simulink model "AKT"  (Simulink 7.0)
settings: Solver=ode45  StartTime=0.0  StopTime=100  RelTol=1e-3

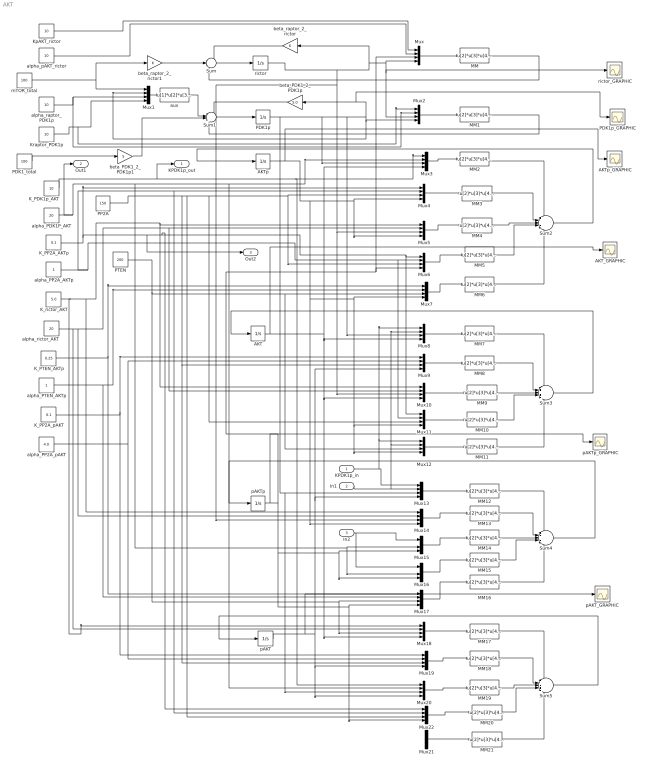
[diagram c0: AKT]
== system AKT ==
  KPDK1p_in : Inport  OutDataType=sfix(16)  OutScaling=2^0
  In1 : Inport  Port=2  OutDataType=sfix(16)  OutScaling=2^0
  In2 : Inport  Port=3  OutDataType=sfix(16)  OutScaling=2^0
  AKT : Integrator  InitialCondition=100.0
  AKT_GRAPHIC : Scope
  AKTp : Integrator  InitialCondition=0.0
  AKTp_GRAPHIC : Scope
  K_PDK1p_AKT : Constant  Value=10  OutDataType=sfix(16)  OutScaling=2^0
  K_PP2A_AKTp : Constant  Value=0.1  OutDataType=sfix(16)  OutScaling=2^0
  K_PP2A_pAKT : Constant  Value=0.1  OutDataType=sfix(16)  OutScaling=2^0
  K_PTEN_AKTp : Constant  Value=0.25  OutDataType=sfix(16)  OutScaling=2^0
  K_rictor_AKT : Constant  Value=5.0  OutDataType=sfix(16)  OutScaling=2^0
  KpAKT_rictor : Constant  Value=10  OutDataType=sfix(16)  OutScaling=2^0
  Kraptor_PDK1p : Constant  Value=10  OutDataType=sfix(16)  OutScaling=2^0
  MM{,1..21} (22 alike) : Fcn  Expr=u[2]*u[3]*u[4]/(u[1]+u[4])
  Mux{,1..22} (23 alike) : Mux
  PDK1_total : Constant  Value=100  OutDataType=sfix(16)  OutScaling=2^0
  PDK1p : Integrator  InitialCondition=50.0
  PDK1p_GRAPHIC : Scope
  PP2A : Constant  Value=150  OutDataType=sfix(16)  OutScaling=2^0
  PTEN : Constant  Value=200  OutDataType=sfix(16)  OutScaling=2^0
  Sum : Sum  Inputs=-+-  OutDataType=sfix(16)  OutScaling=2^0
  Sum1 : Sum  Inputs=--++  OutDataType=sfix(16)  OutScaling=2^0
  Sum2 : Sum  Inputs=+--+-  OutDataType=sfix(16)  OutScaling=2^0
  Sum3 : Sum  Inputs=-+-++  OutDataType=sfix(16)  OutScaling=2^0
  Sum4 : Sum  Inputs=++---  OutDataType=sfix(16)  OutScaling=2^0
  Sum5 : Sum  Inputs=+--++  OutDataType=sfix(16)  OutScaling=2^0
  alpha_PDK1P_AKT : Constant  Value=20  OutDataType=sfix(16)  OutScaling=2^0
  alpha_PP2A_AKTp : Constant  OutDataType=sfix(16)  OutScaling=2^0
  alpha_PP2A_pAKT : Constant  Value=4.0  OutDataType=sfix(16)  OutScaling=2^0
  alpha_PTEN_AKTp : Constant  OutDataType=sfix(16)  OutScaling=2^0
  alpha_pAKT_rictor : Constant  Value=10  OutDataType=sfix(16)  OutScaling=2^0
  alpha_raptor_PDK1p : Constant  Value=10  OutDataType=sfix(16)  OutScaling=2^0
  alpha_rictor_AKT : Constant  Value=20  OutDataType=sfix(16)  OutScaling=2^0
  aux : Fcn  Expr=u[1]*u[2]*u[3]/(u[4]+u[2])
  beta_PDK1_2_PDK1p : Gain  Orientation=left  Gain=5.0  ParameterDataType=sfix(16)  ParameterScaling=2^0  OutDataType=sfix(16)  OutScaling=2^0
  beta_PDK1_2_PDK1p1 : Gain  Gain=5  ParameterDataType=sfix(16)  ParameterScaling=2^0  OutDataType=sfix(16)  OutScaling=2^0
  beta_raptor_2_rictor : Gain  Orientation=left  ParameterDataType=sfix(16)  ParameterScaling=2^0  OutDataType=sfix(16)  OutScaling=2^0
  beta_raptor_2_rictor1 : Gain  ParameterDataType=sfix(16)  ParameterScaling=2^0  OutDataType=sfix(16)  OutScaling=2^0
  mTOR_total : Constant  Value=100  OutDataType=sfix(16)  OutScaling=2^0
  pAKT : Integrator  InitialCondition=.0
  "pAKT_GRAPHIC " : Scope
  pAKTp : Integrator  InitialCondition=0.0
  pAKTp_GRAPHIC : Scope
  rictor : Integrator  InitialCondition=0.0
  rictor_GRAPHIC : Scope
  KPDK1p_out : Outport  OutDataType=sfix(16)  OutScaling=2^0
  Out1 : Outport  Port=2  OutDataType=sfix(16)  OutScaling=2^0
  Out2 : Outport  Port=3  OutDataType=sfix(16)  OutScaling=2^0
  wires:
  Sum/1 -> rictor/1
  rictor/1 -> beta_raptor_2_rictor/1, Mux/4, Mux2/3, rictor_GRAPHIC/1, Mux5/3, Mux10/3, Mux14/3
  beta_raptor_2_rictor/1 -> Sum/1
  beta_raptor_2_rictor1/1 -> Sum/2
  mTOR_total/1 -> beta_raptor_2_rictor1/1, Mux1/1
  Mux/1 -> MM/1
  pAKTp/1 -> Mux/3, Mux6/4, Mux15/4, Mux16/4, Mux17/4, Mux22/4, pAKTp_GRAPHIC/1
  KpAKT_rictor/1 -> Mux/1
  alpha_pAKT_rictor/1 -> Mux/2
  MM/1 -> Sum/3
  Sum1/1 -> PDK1p/1
  PDK1p/1 -> Mux3/3, Mux1/2, Mux2/4, beta_PDK1_2_PDK1p/1, PDK1p_GRAPHIC/1, Mux8/3, Mux13/3, Mux20/3
  beta_PDK1_2_PDK1p/1 -> Sum1/1
  Mux1/1 -> aux/1
  aux/1 -> Sum1/2
  alpha_raptor_PDK1p/1 -> Mux1/3, Mux2/2
  Kraptor_PDK1p/1 -> Mux1/4, Mux2/1
  PDK1_total/1 -> beta_PDK1_2_PDK1p1/1
  beta_PDK1_2_PDK1p1/1 -> Sum1/3
  Mux2/1 -> MM1/1
  MM1/1 -> Sum1/4
  Mux3/1 -> MM2/1
  Mux4/1 -> MM3/1
  Mux5/1 -> MM4/1
  Mux7/1 -> MM6/1
  Mux6/1 -> MM5/1
  MM4/1 -> Sum2/3
  MM3/1 -> Sum2/2
  MM2/1 -> Sum2/1
  MM5/1 -> Sum2/4
  MM6/1 -> Sum2/5
  AKT/1 -> Mux3/4, Mux8/4, Mux10/4, Mux18/4, AKT_GRAPHIC/1
  AKTp/1 -> Mux4/4, Mux5/4, Mux7/4, Mux11/4, Mux12/4, Mux14/4, AKTp_GRAPHIC/1
  Sum2/1 -> AKTp/1
  K_PDK1p_AKT/1 -> Mux20/1, Mux3/1, KPDK1p_out/1
  alpha_PDK1P_AKT/1 -> Mux20/2, Mux3/2, Mux15/3, Mux16/3, Out1/1
  K_PP2A_AKTp/1 -> Mux4/1, Mux22/1, Mux6/1, Mux11/1, Out2/1
  alpha_PP2A_AKTp/1 -> Mux4/2, Mux22/2, Mux6/2, Mux11/2
  PP2A/1 -> Mux9/3, Mux19/3, Mux22/3, Mux4/3, Mux6/3, Mux11/3
  K_rictor_AKT/1 -> Mux5/1, Mux10/1, Mux14/1, Mux18/1
  alpha_rictor_AKT/1 -> Mux5/2, Mux10/2, Mux14/2, Mux18/2
  K_PTEN_AKTp/1 -> Mux17/1, Mux7/1
  alpha_PTEN_AKTp/1 -> Mux17/2, Mux7/2
  PTEN/1 -> Mux17/3, Mux18/3, Mux7/3, Mux12/3
  MM9/1 -> Sum3/3
  MM7/1 -> Sum3/1
  MM8/1 -> Sum3/2
  MM10/1 -> Sum3/4
  MM11/1 -> Sum3/5
  Sum3/1 -> AKT/1
  Mux8/1 -> MM7/1
  Mux9/1 -> MM8/1
  Mux10/1 -> MM9/1
  Mux11/1 -> MM10/1
  Mux12/1 -> MM11/1
  K_PP2A_pAKT/1 -> Mux9/1, Mux19/1
  alpha_PP2A_pAKT/1 -> Mux9/2, Mux19/2
  pAKT/1 -> Mux9/4, Mux13/4, Mux19/4, Mux20/4, "pAKT_GRAPHIC "/1
  MM14/1 -> Sum4/3
  MM12/1 -> Sum4/1
  MM13/1 -> Sum4/2
  MM15/1 -> Sum4/4
  MM16/1 -> Sum4/5
  Sum4/1 -> pAKTp/1
  Mux13/1 -> MM12/1
  Mux14/1 -> MM13/1
  Mux15/1 -> MM14/1
  Mux16/1 -> MM15/1
  Mux17/1 -> MM16/1
  MM17/1 -> Sum5/1
  MM18/1 -> Sum5/2
  MM19/1 -> Sum5/3
  MM20/1 -> Sum5/4
  MM21/1 -> Sum5/5
  Mux18/1 -> MM17/1
  Mux19/1 -> MM18/1
  Mux20/1 -> MM19/1
  Mux22/1 -> MM20/1
  Mux21/1 -> MM21/1
  Sum5/1 -> pAKT/1
  KPDK1p_in/1 -> Mux13/1, Mux8/1, Mux12/1
  In1/1 -> Mux13/2, Mux8/2, Mux12/2
  In2/1 -> Mux15/1, Mux16/1
